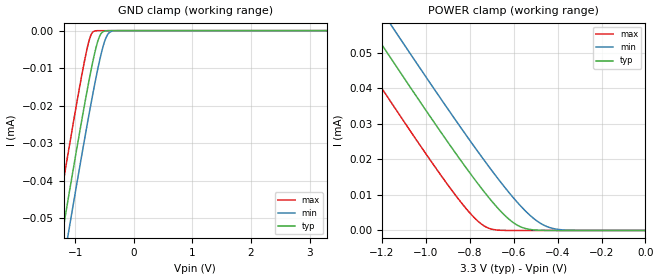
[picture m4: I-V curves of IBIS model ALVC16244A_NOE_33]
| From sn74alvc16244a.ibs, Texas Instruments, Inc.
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[Model]   ALVC16244A_NOE_33
Model_type  Input
Vinl=0.8
Vinh=2.0
| variable   typ   min   max
C_comp   0.78pF   0.48pF   0.96pF
[Temperature Range]   40   100   -40
| Ambient temperature   25   85   -40
[Voltage range]   3.3   3   3.6
[GND Clamp]
| ALVC16244A_NOE_33
|   Voltage   I(typ)   I(min)   I(max)
-3.3V     -253.6uA   -262.7uA   -242uA
-1.385V   -69.59uA   -79.01uA   -57.34uA
-1.33V    -64.41uA   -73.84uA   -52.15uA
-1.23V    -55.05uA   -64.49uA   -42.75uA
-1.105V   -43.45uA   -52.89uA   -31.15uA
-815mV    -17.51uA   -26.69uA   -6.053uA
-745mV    -11.74uA   -20.66uA   -1.726uA
-680mV    -6.833uA   -15.27uA   -159.4nA
-590mV    -1.733uA   -8.391uA   -2.178nA
-505mV    -143.8nA   -3.188uA   -43.3pA
-370mV    -1.152nA   -136.1nA   -8.019pA
3.3V      6.303pA    16.85nA    5.63pA
[POWER Clamp]
| ALVC16244A_NOE_33
|   Voltage   I(typ)   I(min)   I(max)
-3.3V     253.6uA    262.7uA    242uA
-1.39V    70.06uA    79.48uA    57.81uA
-1.27V    58.79uA    68.22uA    46.5uA
-1.215V   53.65uA    63.09uA    41.35uA
-1.165V   49uA       58.44uA    36.7uA
-1.12V    44.83uA    54.27uA    32.53uA
-790mV    15.41uA    24.52uA    4.296uA
-710mV    9.02uA     17.73uA    561.4nA
-600mV    2.14uA     9.107uA    3.534nA
-505mV    143.8nA    3.188uA    43.3pA
-420mV    6.983nA    547nA      8.704pA
-48.03fV  6.303pA    7.801pA    6.677pA
